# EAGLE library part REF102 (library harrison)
Texas Instruments REF102 +10V voltage reference
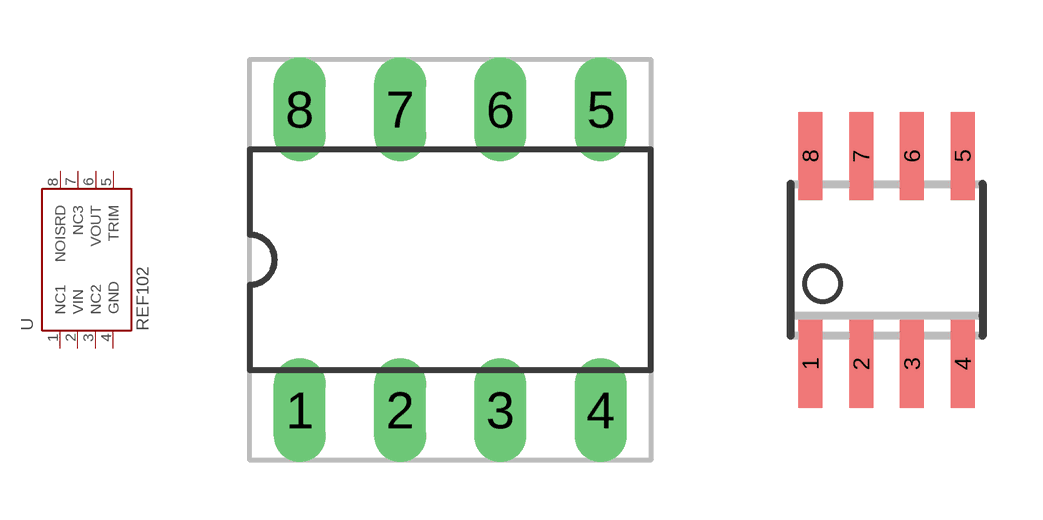
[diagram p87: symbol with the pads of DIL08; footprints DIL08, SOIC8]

Designator prefix U

## REF102-DIP  [DIL08]
1  NC1  nc
2  VIN  pwr
3  NC2  nc
4  GND  pwr
5  TRIM  in
6  VOUT  out
7  NC3  nc
8  NOISRD  pas

## REF102-SOIC  [SOIC8]
Pads as for DIL08

## Footprint DIL08 (pad centres in mm)
drill 0.813 long: 1 -3.81,-3.81; 2 -1.27,-3.81; 3 1.27,-3.81; 4 3.81,-3.81; 5 3.81,3.81; 6 1.27,3.81; 7 -1.27,3.81; 8 -3.81,3.81

## Footprint SOIC8 (pad centres in mm)
smd 0.6 x 2.2: 1 -1.905,-2.6; 2 -0.635,-2.6; 3 0.635,-2.6; 4 1.905,-2.6; 5 1.905,2.6; 6 0.635,2.6; 7 -0.635,2.6; 8 -1.905,2.6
